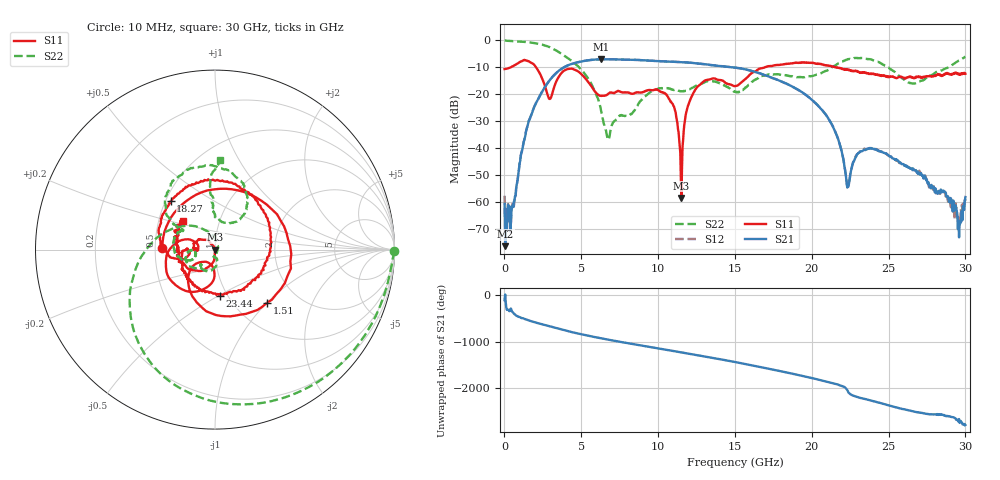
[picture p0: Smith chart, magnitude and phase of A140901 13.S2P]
!  2-Port S-parameters saved by WinCal
! VAR MeasName=S-Parameters (CALIBRATED_DATA) read from VNA (N5244A)
! VAR MeasDate=11/3/2014 9:27:46 AM
! VAR NAME=A140901 13
! VAR FILENAME=A140901 13.S2P
! VAR DATE=11/3/2014 9:27:46 AM
! VAR PHYS_PORTS=1,2
# Hz S RI R 50
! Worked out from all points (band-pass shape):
!   801 points, 10 MHz to 30 GHz, reference 50 ohm
!   highest |S21| = -6.97 dB at 6.308 GHz (marker M1); lowest = -76.4 dB at 47.49 MHz (marker M2)
!   |S21| within 3 dB of the highest: 3.871 GHz to 14.81 GHz (10.94 GHz wide, 117 % of centre)
!   lowest |S11| = -58.5 dB at 11.52 GHz (marker M3), VSWR 1.00, Z = 50.1 + j0.0542 ohm
!   |S11| at or under -10 dB: start of sweep to 404.7 MHz; 2.055 GHz to 16.94 GHz (14.89 GHz wide, 157 % of centre); 21.64 GHz to end of sweep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
!   |S22| runs from -36.9 to 0.0 dB; largest |S21 - S12| = 0.0023
!   S11 on the Smith chart (normalised r, x): 10 MHz: 0.55, +0.01; 1.51 GHz: 1.40, -1.00; 18.27 GHz: 0.53, +0.33; 23.44 GHz: 0.92, -0.51; 30 GHz: 0.67, +0.23
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1e7  -0.2933 0.00755  -0.000357 -0.000857  -0.000371 0.00126  0.9983 -0.00867
4.74875e7  -0.2925 0.0363  0.000151 1.75e-05  -0.000309 1.08e-06  0.9932 -0.0375
4.5985e8  -0.1064 0.3053  0.000594 0.000391  0.000659 0.000444  0.93 -0.2874
1.5095e9  0.2896 -0.2965  -0.0263 -0.00165  -0.0264 -0.0016  0.5208 -0.7672
2.934025e9  -0.0386 -0.0722  0.1233 0.1326  0.1229 0.1325  -0.3125 -0.6828
5.033325e9  -0.231 0.0256  -0.2339 -0.3361  -0.2339 -0.3361  -0.2603 0.1056
6.3079e9  -0.093 0.00699  -0.385 0.2298  -0.385 0.2294  0.00508 0.0468
6.75775e9  -0.1024 -0.00576  -0.2314 0.3838  -0.2316 0.3832  0.0137 -0.00425
8.519662e9  -0.1068 0.00446  0.4148 0.1328  0.4148 0.1329  0.0111 -0.0528
1.001916e10  -0.1137 0.0374  0.1636 -0.3801  0.1627 -0.3792  -0.0466 -0.1192
1.099384e10  -0.0352 0.0504  -0.207 -0.3441  -0.2067 -0.3441  -0.0801 -0.0899
1.151866e10  0.00106 0.000541  -0.3455 -0.192  -0.3445 -0.1918  -0.0781 -0.0819
1.249334e10  -0.0643 -0.1139  -0.3335 0.1737  -0.3341 0.1741  -0.1036 -0.1037
1.5005e10  -0.1409 -0.0166  0.3122 0.021  0.3119 0.0201  -0.1103 -0.0124
1.826641e10  -0.2472 0.2688  -0.1352 0.0888  -0.1352 0.0882  -0.2058 0.0938
2.002832e10  0.0935 0.3734  0.0741 0.0247  0.0741 0.0252  -0.1864 0.1109
2.149034e10  0.3088 0.0795  -0.00373 -0.0213  -0.00346 -0.0213  -0.272 0.2027
2.235255e10  0.2561 -0.1321  -0.000315 0.00192  -0.000306 0.00192  -0.2383 0.3825
2.343969e10  0.0273 -0.256  0.00383 -0.00849  0.00375 -0.00911  0.00149 0.464
2.501416e10  -0.1675 -0.1222  -0.00658 0.00308  -0.00652 0.00304  0.1808 0.2545
2.958764e10  -0.1871 0.1371  -0.000161 -0.000152  -0.000256 0.000256  -0.0176 0.4225
3e10  -0.1793 0.1602  -0.000119 0.00124  0.000158 0.00104  0.0294 0.4966
